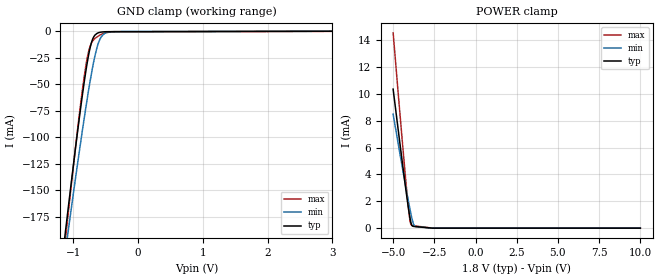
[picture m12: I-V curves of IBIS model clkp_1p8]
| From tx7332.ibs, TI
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|   clkp_1p8 Model
[Model]   clkp_1p8
Model_type   Input
Vinl = 0.45
Vinh = 1.35
|   typ   min   max
C_comp   10.512pF   9.676pF   10.956pF
[Model spec]
|subparameter
Vinl   0.45   0.425   0.475
Vinh   1.35   1.275   1.425
| Where Nom  PVT is Nominal Process, 1.8V, 27C
|   Fast PVT is Strong Process,  1.9V, 0C
|   Slow PVT is Weak Process,   1.7V, 100C
[Voltage Range]   1.8   1.7   1.9
|Junction Temperature
[Temperature Range]   27   100   0
[Power Clamp Reference]   1.8   1.7   1.9
[GND Clamp Reference]   0   0   0
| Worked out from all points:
|   GND clamp passes 1 mA (typ) near -0.58 V on its own axis
|   POWER clamp passes 1 mA (typ) near -4.01 V on its own axis
[GND Clamp]
|   Voltage   I(typ)   I(min)   I(max)
-5V       -2.315A    -2.046A    -2.569A
-1.13V    -192.6mA   -210.6mA   -200.3mA
-1.1V     -177.1mA   -197.1mA   -183.2mA
-1.07V    -161.7mA   -183.8mA   -166.2mA
-905mV    -80.27mA   -111.9mA   -76.85mA
-800mV    -34.8mA    -69.04mA   -29.89mA
-755mV    -19.39mA   -51.99mA   -16.83mA
-710mV    -8.793mA   -36.32mA   -10.05mA
-590mV    -1.16mA    -7.64mA    -3.743mA
-515mV    -650.1uA   -2.162mA   -1.741mA
-365mV    -545.5uA   -524.1uA   -778.9uA
10V       0A         0A         0A
[POWER Clamp]
|   Voltage   I(typ)   I(min)   I(max)
-5V       10.35mA    8.489mA    14.54mA
-4.46V    5.07mA     4.651mA    6.719mA
-4.16V    2.263mA    2.588mA    2.593mA
-4.07V    1.482mA    1.994mA    1.484mA
-3.995V   891.6uA    1.516mA    718uA
-3.95V    587.3uA    1.241mA    404.8uA
-3.89V    290.1uA    895.3uA    228.5uA
-3.83V    162.7uA    585.5uA    195.1uA
-3.755V   131.5uA    287.8uA    181.2uA
-3.65V    118.1uA    120.8uA    164.6uA
-2.63V    1.743uA    321.8nA    4.306uA
10V       0A         0A         0A
